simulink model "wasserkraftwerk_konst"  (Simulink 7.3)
settings: Solver=ode23tb  StartTime=0.0  StopTime=1000  MaxStep=0.1  RelTol=1e-4
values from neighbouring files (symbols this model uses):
  A_V0 = 0.518    [Parameter_sim.m]
  A_W = 5^2*pi    (= 78.5398163397)    [Parameter_sim.m]
  c_d = 0.9658    [Parameter_sim.m]
  d_F = 2    [Parameter_sim.m]
  d_T = 3    [Parameter_sim.m]
  d_Turb = 5.35    [Parameter_sim.m]
  g = 9.81    [Parameter_sim.m]
  h_R = 413    [Parameter_sim.m]
  h_W0 = 390    [Parameter_sim.m]
  h_W_IC = 413    [Parameter_sim.m]
  I_IC = 0    [Parameter_sim.m]
  kappa = 8.7*10^3    (= 8700)    [Parameter_sim.m]
  l_F = 741    [Parameter_sim.m]
  L_G = 0.1    [Parameter_sim.m]
  L_net = 0.1    [Parameter_sim.m]
  l_T = 2000    [Parameter_sim.m]
  lambda_F = 0.0153    [Parameter_sim.m]
  lambda_T = 0.0182    [Parameter_sim.m]
  lambda_W = 4.0738    [Parameter_sim.m]
  omega_IC = 0    [Parameter_sim.m]
  p_0 = 0    [Parameter_sim.m]
  R_G = 10    [Parameter_sim.m]
  R_net = 165    [Parameter_sim.m]
  rho = 1000    [Parameter_sim.m]
  sigma_0 = 6.2790e-010    (= 6.279e-10)    [Parameter_sim.m]
  Theta = 5.4997*10^3    (= 5499.7)    [Parameter_sim.m]
  v_F_IC = 0    [Parameter_sim.m]
  V_F_IC = l_F*pi*d_F^2/4    (= 2327.92015631)    [Parameter_sim.m]
  v_T_IC = 0    [Parameter_sim.m]

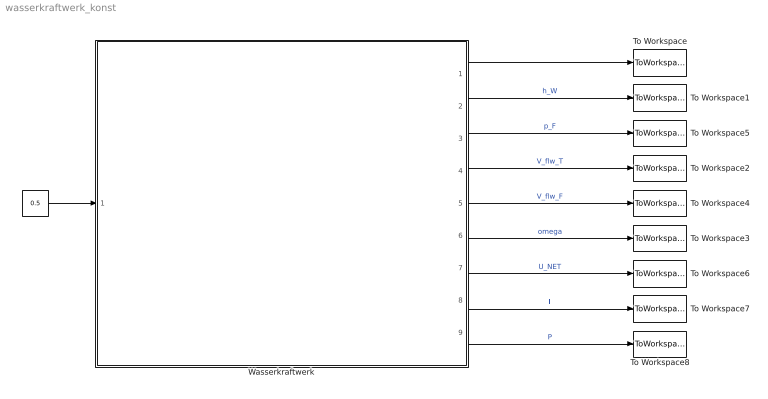
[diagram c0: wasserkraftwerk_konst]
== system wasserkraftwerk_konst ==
  " " : Constant  Value=0.5  OutDataType=sfix(16)  OutScaling=2^0
  To Workspace : ToWorkspace  VariableName=x  SampleTime=-1  SaveFormat=Array
  To Workspace1 : ToWorkspace  VariableName=h_W  SampleTime=-1  SaveFormat=Array
  To Workspace2 : ToWorkspace  VariableName=V_flw_T  SampleTime=-1  SaveFormat=Array
  To Workspace3 : ToWorkspace  VariableName=omega  SampleTime=-1  SaveFormat=Array
  To Workspace4 : ToWorkspace  VariableName=V_flw_F  SampleTime=-1  SaveFormat=Array
  To Workspace5 : ToWorkspace  VariableName=p_F  SampleTime=-1  SaveFormat=Array
  To Workspace6 : ToWorkspace  VariableName=U_NET  SampleTime=-1  SaveFormat=Array
  To Workspace7 : ToWorkspace  VariableName=I  SampleTime=-1  SaveFormat=Array
  To Workspace8 : ToWorkspace  VariableName=P  SampleTime=-1  SaveFormat=Array
  Wasserkraftwerk : Subsystem
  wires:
  " "/1 -> Wasserkraftwerk/1(in)
  Wasserkraftwerk/1(x) -> To Workspace/1
  Wasserkraftwerk/2(h_W) -> To Workspace1/1  "h_W"
  Wasserkraftwerk/3(p_F) -> To Workspace5/1  "p_F"
  Wasserkraftwerk/4(V_flw_T) -> To Workspace2/1  "V_flw_T"
  Wasserkraftwerk/5(V_flw_F) -> To Workspace4/1  "V_flw_F"
  Wasserkraftwerk/6(omega) -> To Workspace3/1  "omega"
  Wasserkraftwerk/7(U_NET) -> To Workspace6/1  "U_NET"
  Wasserkraftwerk/8(I) -> To Workspace7/1  "I"
  Wasserkraftwerk/9(P) -> To Workspace8/1  "P"

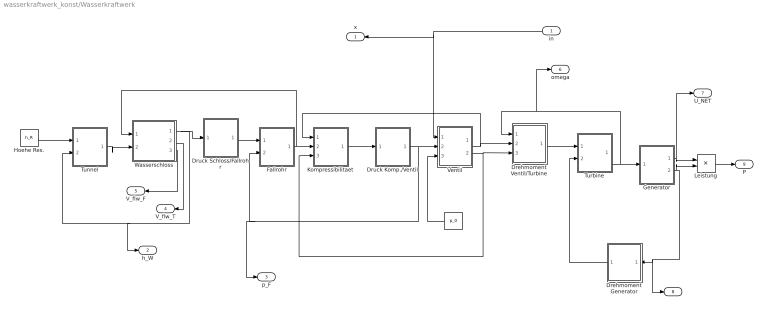
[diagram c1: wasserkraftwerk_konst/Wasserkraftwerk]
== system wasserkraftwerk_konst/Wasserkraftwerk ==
  in : Inport  OutDataType=sfix(16)  OutScaling=2^0
  " " : Constant  Value=p_0  OutDataType=sfix(16)  OutScaling=2^0
  Drehmoment Generator : Subsystem
  Drehmoment Ventil/Turbine : Subsystem
  Druck Komp./Ventil : Subsystem
  Druck Schloss/Fallrohr : Subsystem
  Fallrohr : Subsystem
  Generator : Subsystem
  Hoehe Res. : Constant  Value=h_R  OutDataType=sfix(16)  OutScaling=2^0
  Kompressibilitaet : Subsystem
  Leistung : Product  OutDataType=sfix(16)  OutScaling=2^0
  Tunnel : Subsystem
  Turbine : Subsystem
  Ventil : Subsystem
  Wasserschloss : Subsystem
  x : Outport  OutDataType=sfix(16)  OutScaling=2^0
  h_W : Outport  Port=2  OutDataType=sfix(16)  OutScaling=2^0
  p_F : Outport  Port=3  OutDataType=sfix(16)  OutScaling=2^0
  V_flw_T : Outport  Port=4  OutDataType=sfix(16)  OutScaling=2^0
  V_flw_F : Outport  Port=5  OutDataType=sfix(16)  OutScaling=2^0
  omega : Outport  Port=6  OutDataType=sfix(16)  OutScaling=2^0
  U_NET : Outport  Port=7  OutDataType=sfix(16)  OutScaling=2^0
  I : Outport  Port=8  OutDataType=sfix(16)  OutScaling=2^0
  P : Outport  Port=9  OutDataType=sfix(16)  OutScaling=2^0
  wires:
  Hoehe Res./1 -> Tunnel/1(h_R)
  Tunnel/1(v_T) -> Wasserschloss/2(v_T)
  Wasserschloss/1(h_W) -> Druck Schloss/Fallrohr/1(h_W), Tunnel/2(h_W), h_W/1
  Druck Schloss/Fallrohr/1(p_W) -> Fallrohr/1(p_W)
  Fallrohr/1(v_F) -> Kompressibilitaet/2(v_F), Wasserschloss/1(v_F)
  Kompressibilitaet/1(V) -> Druck Komp./Ventil/1(V)
  Druck Komp./Ventil/1(p_F) -> Ventil/2(p_F), Fallrohr/2(p_F), p_F/1
  Ventil/1(A_V) -> Drehmoment Ventil/Turbine/2(A_V), Kompressibilitaet/1(A_V)
  Drehmoment Ventil/Turbine/1(T_T) -> Turbine/1(T_T)
  Turbine/1(w) -> Generator/1(w), Drehmoment Ventil/Turbine/1(w), omega/1
  Generator/2(I) -> Drehmoment Generator/1(I), I/1, Leistung/2
  Ventil/2(v_V) -> Drehmoment Ventil/Turbine/3(v_V), Kompressibilitaet/3(v_V)
  Generator/1(U_NET) -> U_NET/1, Leistung/1
  Leistung/1 -> P/1
  Wasserschloss/2(V_flw_T) -> V_flw_T/1
  Wasserschloss/3(V_flw_F) -> V_flw_F/1
  " "/1 -> Ventil/3(p_0)
  Drehmoment Generator/1(T_G) -> Turbine/2(T_G)
  in/1 -> Ventil/1(x), x/1

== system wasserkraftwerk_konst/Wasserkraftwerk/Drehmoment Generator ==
  I : Inport  OutDataType=sfix(16)  OutScaling=2^0
  Gain : Gain  Gain=kappa  ParameterDataType=sfix(16)  ParameterScaling=2^0  OutDataType=sfix(16)  OutScaling=2^0
  T_G : Outport  OutDataType=sfix(16)  OutScaling=2^0
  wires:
  I/1 -> Gain/1
  Gain/1 -> T_G/1

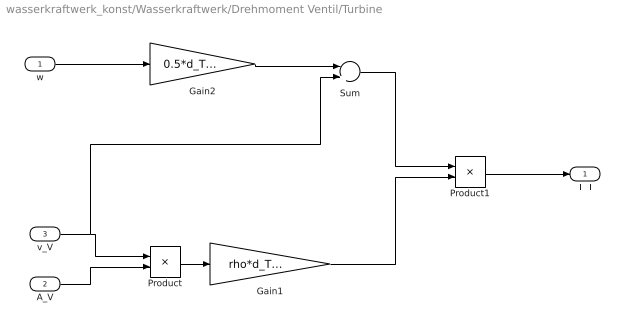
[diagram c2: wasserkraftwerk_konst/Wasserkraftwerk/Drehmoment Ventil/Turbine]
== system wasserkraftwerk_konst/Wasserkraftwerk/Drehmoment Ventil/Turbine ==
  w : Inport  OutDataType=sfix(16)  OutScaling=2^0
  A_V : Inport  Port=2  OutDataType=sfix(16)  OutScaling=2^0
  v_V : Inport  Port=3  OutDataType=sfix(16)  OutScaling=2^0
  Gain1 : Gain  Gain=rho*d_Turb  ParameterDataType=sfix(16)  ParameterScaling=2^0  OutDataType=sfix(16)  OutScaling=2^0
  Gain2 : Gain  Gain=0.5*d_Turb  ParameterDataType=sfix(16)  ParameterScaling=2^0  OutDataType=sfix(16)  OutScaling=2^0
  Product : Product  OutDataType=sfix(16)  OutScaling=2^0
  Product1 : Product  OutDataType=sfix(16)  OutScaling=2^0
  Sum : Sum  Inputs=-+  OutDataType=sfix(16)  OutScaling=2^0
  T_T : Outport  OutDataType=sfix(16)  OutScaling=2^0
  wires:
  Product/1 -> Gain1/1
  w/1 -> Gain2/1
  Gain2/1 -> Sum/1
  v_V/1 -> Product/1, Sum/2
  A_V/1 -> Product/2
  Sum/1 -> Product1/1
  Gain1/1 -> Product1/2
  Product1/1 -> T_T/1

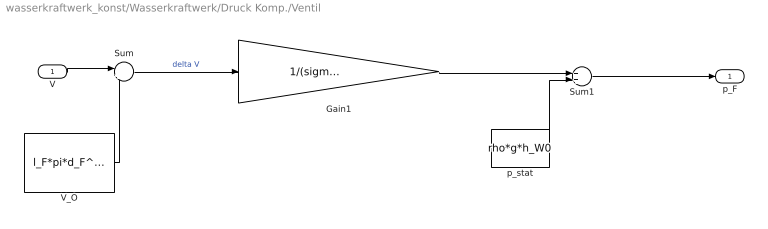
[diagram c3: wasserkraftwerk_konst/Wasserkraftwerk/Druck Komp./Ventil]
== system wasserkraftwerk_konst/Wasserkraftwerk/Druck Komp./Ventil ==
  V : Inport  OutDataType=sfix(16)  OutScaling=2^0
  Gain1 : Gain  Gain=1/(sigma_0 * l_F*pi*d_F^2/4)  ParameterDataType=sfix(16)  ParameterScaling=2^0  OutDataType=sfix(16)  OutScaling=2^0
  Sum : Sum  Inputs=|+-  OutDataType=sfix(16)  OutScaling=2^0
  Sum1 : Sum  OutDataType=sfix(16)  OutScaling=2^0
  V_O : Constant  Value=l_F*pi*d_F^2/4  OutDataType=sfix(16)  OutScaling=2^0
  p_stat : Constant  Value=rho*g*h_W0  OutDataType=sfix(16)  OutScaling=2^0
  p_F : Outport  OutDataType=sfix(16)  OutScaling=2^0
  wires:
  V/1 -> Sum/1
  V_O/1 -> Sum/2
  Sum1/1 -> p_F/1
  p_stat/1 -> Sum1/2
  Sum/1 -> Gain1/1  "delta V"
  Gain1/1 -> Sum1/1

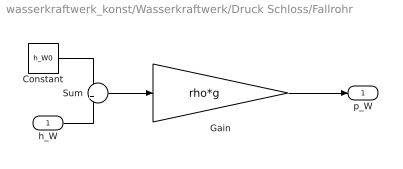
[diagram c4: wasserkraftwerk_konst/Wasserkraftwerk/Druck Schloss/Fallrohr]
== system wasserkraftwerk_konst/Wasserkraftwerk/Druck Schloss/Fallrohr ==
  h_W : Inport  OutDataType=sfix(16)  OutScaling=2^0
  Constant : Constant  Value=h_W0  OutDataType=sfix(16)  OutScaling=2^0
  Gain : Gain  Gain=rho*g  ParameterDataType=sfix(16)  ParameterScaling=2^0  OutDataType=sfix(16)  OutScaling=2^0
  Sum : Sum  Inputs=-+  OutDataType=sfix(16)  OutScaling=2^0
  p_W : Outport  OutDataType=sfix(16)  OutScaling=2^0
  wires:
  Gain/1 -> p_W/1
  Constant/1 -> Sum/1
  h_W/1 -> Sum/2
  Sum/1 -> Gain/1

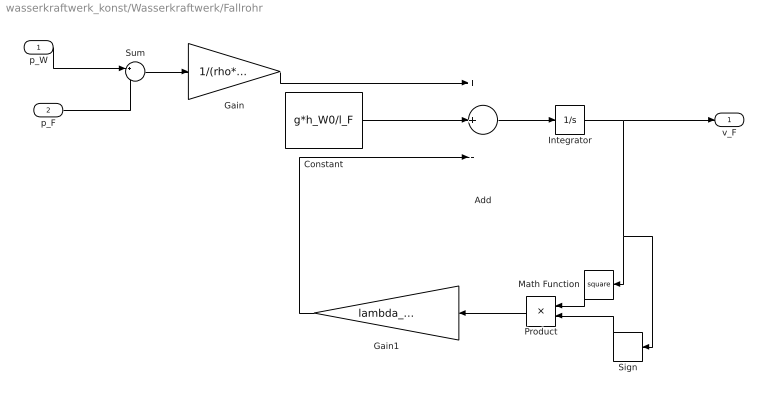
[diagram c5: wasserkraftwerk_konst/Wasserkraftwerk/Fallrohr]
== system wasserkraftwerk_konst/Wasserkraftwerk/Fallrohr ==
  p_W : Inport  OutDataType=sfix(16)  OutScaling=2^0
  p_F : Inport  Port=2  OutDataType=sfix(16)  OutScaling=2^0
  Add : Sum  Inputs=++-  OutDataType=sfix(16)  OutScaling=2^-10
  Constant : Constant  Value=g*h_W0/l_F  OutDataType=sfix(16)  OutScaling=2^0
  Gain : Gain  Gain=1/(rho*l_F)  ParameterDataType=sfix(16)  ParameterScaling=2^0  OutDataType=sfix(16)  OutScaling=2^0
  Gain1 : Gain  Gain=lambda_F/(2*d_F)  ParameterDataType=sfix(16)  ParameterScaling=2^0  OutDataType=sfix(16)  OutScaling=2^0
  Integrator : Integrator  InitialCondition=v_F_IC
  Math Function : Math  Operator=square  OutDataType=sfix(16)  OutScaling=2^0
  Product : Product  OutDataType=sfix(16)  OutScaling=2^0
  Sign : Signum
  Sum : Sum  Inputs=+-  OutDataType=sfix(16)  OutScaling=2^0
  v_F : Outport  OutDataType=sfix(16)  OutScaling=2^0
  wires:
  Product/1 -> Gain1/1
  Sign/1 -> Product/2
  p_W/1 -> Sum/1
  p_F/1 -> Sum/2
  Sum/1 -> Gain/1
  Gain/1 -> Add/1
  Gain1/1 -> Add/3
  Add/1 -> Integrator/1
  Integrator/1 -> v_F/1, Math Function/1, Sign/1
  Math Function/1 -> Product/1
  Constant/1 -> Add/2

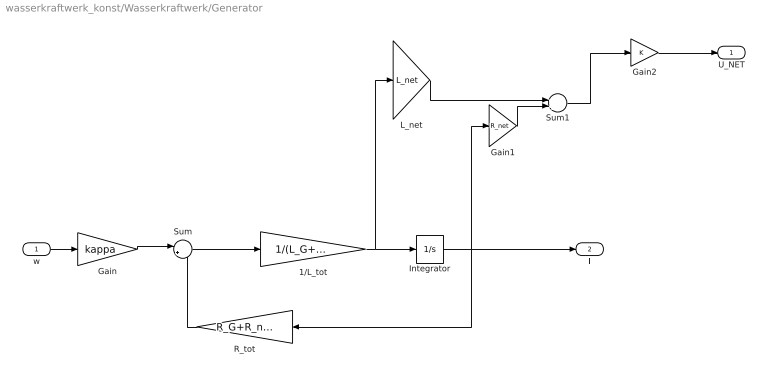
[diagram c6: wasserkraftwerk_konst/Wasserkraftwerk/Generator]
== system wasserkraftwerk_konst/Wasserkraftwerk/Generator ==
  w : Inport  OutDataType=sfix(16)  OutScaling=2^0
  1/L_tot : Gain  Gain=1/(L_G+L_net)  ParameterDataType=sfix(16)  ParameterScaling=2^0  OutDataType=sfix(16)  OutScaling=2^0
  Gain : Gain  Gain=kappa  ParameterDataType=sfix(16)  ParameterScaling=2^0  OutDataType=sfix(16)  OutScaling=2^0
  Gain1 : Gain  Gain=R_net  ParameterDataType=sfix(16)  ParameterScaling=2^0  OutDataType=sfix(16)  OutScaling=2^0
  Gain2 : Gain  ParameterDataType=sfix(16)  ParameterScaling=2^0  OutDataType=sfix(16)  OutScaling=2^0
  Integrator : Integrator  InitialCondition=I_IC
  L_net : Gain  Gain=L_net  ParameterDataType=sfix(16)  ParameterScaling=2^0  OutDataType=sfix(16)  OutScaling=2^0
  R_tot : Gain  Gain=R_G+R_net  ParameterDataType=sfix(16)  ParameterScaling=2^0  OutDataType=sfix(16)  OutScaling=2^0
  Sum : Sum  Inputs=|+-  OutDataType=sfix(16)  OutScaling=2^0
  Sum1 : Sum  OutDataType=sfix(16)  OutScaling=2^0
  U_NET : Outport  OutDataType=sfix(16)  OutScaling=2^0
  I : Outport  Port=2  OutDataType=sfix(16)  OutScaling=2^0
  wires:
  Integrator/1 -> I/1, R_tot/1, Gain1/1
  w/1 -> Gain/1
  Gain/1 -> Sum/1
  Sum/1 -> 1/L_tot/1
  1/L_tot/1 -> Integrator/1, L_net/1
  Gain2/1 -> U_NET/1
  Gain1/1 -> Sum1/2
  R_tot/1 -> Sum/2
  Sum1/1 -> Gain2/1
  L_net/1 -> Sum1/1

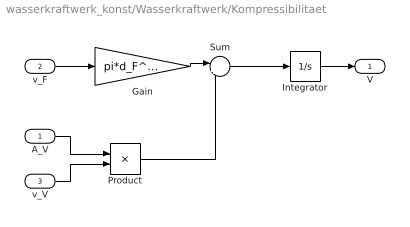
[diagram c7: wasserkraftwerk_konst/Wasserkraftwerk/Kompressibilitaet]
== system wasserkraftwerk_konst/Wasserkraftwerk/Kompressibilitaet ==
  A_V : Inport  OutDataType=sfix(16)  OutScaling=2^0
  v_F : Inport  Port=2  OutDataType=sfix(16)  OutScaling=2^0
  v_V : Inport  Port=3  OutDataType=sfix(16)  OutScaling=2^0
  Gain : Gain  Gain=pi*d_F^2/4  ParameterDataType=sfix(16)  ParameterScaling=2^0  OutDataType=sfix(16)  OutScaling=2^0
  Integrator : Integrator  InitialCondition=V_F_IC
  Product : Product  OutDataType=sfix(16)  OutScaling=2^0
  Sum : Sum  Inputs=|+-  OutDataType=sfix(16)  OutScaling=2^0
  V : Outport  OutDataType=sfix(16)  OutScaling=2^0
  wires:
  v_F/1 -> Gain/1
  Gain/1 -> Sum/1
  A_V/1 -> Product/1
  v_V/1 -> Product/2
  Product/1 -> Sum/2
  Sum/1 -> Integrator/1
  Integrator/1 -> V/1

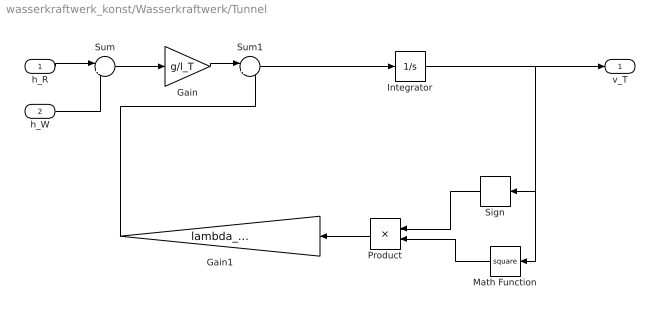
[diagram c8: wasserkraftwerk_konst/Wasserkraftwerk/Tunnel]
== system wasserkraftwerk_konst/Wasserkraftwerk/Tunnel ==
  h_R : Inport  OutDataType=sfix(16)  OutScaling=2^0
  h_W : Inport  Port=2  OutDataType=sfix(16)  OutScaling=2^0
  Gain : Gain  Gain=g/l_T  ParameterDataType=sfix(16)  ParameterScaling=2^0  OutDataType=sfix(16)  OutScaling=2^0
  Gain1 : Gain  Gain=lambda_T/(2*d_T)  ParameterDataType=sfix(16)  ParameterScaling=2^0  OutDataType=sfix(16)  OutScaling=2^0
  Integrator : Integrator  InitialCondition=v_T_IC
  Math Function : Math  Operator=square  OutDataType=sfix(16)  OutScaling=2^0
  Product : Product  OutDataType=sfix(16)  OutScaling=2^0
  Sign : Signum
  Sum : Sum  Inputs=|+-  OutDataType=sfix(16)  OutScaling=2^0
  Sum1 : Sum  Inputs=|+-  OutDataType=sfix(16)  OutScaling=2^0
  v_T : Outport  OutDataType=sfix(16)  OutScaling=2^0
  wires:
  h_R/1 -> Sum/1
  h_W/1 -> Sum/2
  Sum/1 -> Gain/1
  Gain/1 -> Sum1/1
  Sum1/1 -> Integrator/1
  Integrator/1 -> v_T/1, Sign/1, Math Function/1
  Product/1 -> Gain1/1
  Sign/1 -> Product/1
  Math Function/1 -> Product/2
  Gain1/1 -> Sum1/2

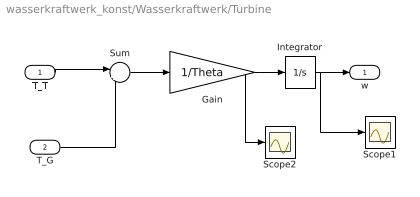
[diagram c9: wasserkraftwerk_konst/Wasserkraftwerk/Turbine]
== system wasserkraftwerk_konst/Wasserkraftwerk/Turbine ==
  T_T : Inport  OutDataType=sfix(16)  OutScaling=2^0
  T_G : Inport  Port=2  OutDataType=sfix(16)  OutScaling=2^0
  Gain : Gain  Gain=1/Theta  ParameterDataType=sfix(16)  ParameterScaling=2^0  OutDataType=sfix(16)  OutScaling=2^0
  Integrator : Integrator  InitialCondition=omega_IC
  Scope1 : Scope
  Scope2 : Scope
  Sum : Sum  Inputs=|+-  OutDataType=sfix(16)  OutScaling=2^0
  w : Outport  OutDataType=sfix(16)  OutScaling=2^0
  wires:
  T_T/1 -> Sum/1
  T_G/1 -> Sum/2
  Sum/1 -> Gain/1
  Gain/1 -> Integrator/1, Scope2/1
  Integrator/1 -> w/1, Scope1/1

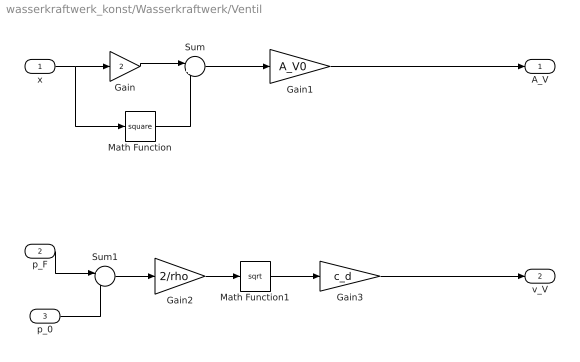
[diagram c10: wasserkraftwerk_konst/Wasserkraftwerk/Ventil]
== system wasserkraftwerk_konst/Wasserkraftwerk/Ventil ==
  x : Inport  OutDataType=sfix(16)  OutScaling=2^0
  p_F : Inport  Port=2  OutDataType=sfix(16)  OutScaling=2^0
  p_0 : Inport  Port=3  OutDataType=sfix(16)  OutScaling=2^0
  Gain : Gain  Gain=2  ParameterDataType=sfix(16)  ParameterScaling=2^0  OutDataType=sfix(16)  OutScaling=2^0
  Gain1 : Gain  Gain=A_V0  ParameterDataType=sfix(16)  ParameterScaling=2^0  OutDataType=sfix(16)  OutScaling=2^0
  Gain2 : Gain  Gain=2/rho  ParameterDataType=sfix(16)  ParameterScaling=2^0  OutDataType=sfix(16)  OutScaling=2^0
  Gain3 : Gain  Gain=c_d  ParameterDataType=sfix(16)  ParameterScaling=2^0  OutDataType=sfix(16)  OutScaling=2^0
  Math Function : Math  Operator=square  OutDataType=sfix(16)  OutScaling=2^0
  Math Function1 : Math  Operator=sqrt  OutDataType=sfix(16)  OutScaling=2^0
  Sum : Sum  Inputs=|+-  OutDataType=sfix(16)  OutScaling=2^0
  Sum1 : Sum  Inputs=+-  OutDataType=sfix(16)  OutScaling=2^0
  A_V : Outport  OutDataType=sfix(16)  OutScaling=2^0
  v_V : Outport  Port=2  OutDataType=sfix(16)  OutScaling=2^0
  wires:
  x/1 -> Gain/1, Math Function/1
  Gain/1 -> Sum/1
  Math Function/1 -> Sum/2
  Sum/1 -> Gain1/1
  Gain1/1 -> A_V/1
  p_F/1 -> Sum1/1
  p_0/1 -> Sum1/2
  Sum1/1 -> Gain2/1
  Gain2/1 -> Math Function1/1
  Math Function1/1 -> Gain3/1
  Gain3/1 -> v_V/1

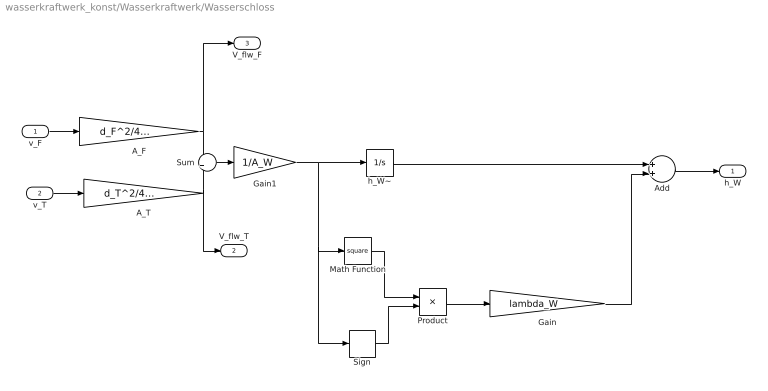
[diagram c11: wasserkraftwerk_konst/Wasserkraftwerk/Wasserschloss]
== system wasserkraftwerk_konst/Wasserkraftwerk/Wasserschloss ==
  v_F : Inport  OutDataType=sfix(16)  OutScaling=2^0
  v_T : Inport  Port=2  OutDataType=sfix(16)  OutScaling=2^0
  A_F : Gain  Gain=d_F^2/4*pi  ParameterDataType=sfix(16)  ParameterScaling=2^0  OutDataType=sfix(16)  OutScaling=2^0
  A_T : Gain  Gain=d_T^2/4*pi  ParameterDataType=sfix(16)  ParameterScaling=2^0  OutDataType=sfix(16)  OutScaling=2^0
  Add : Sum  OutDataType=sfix(16)  OutScaling=2^-10
  Gain : Gain  Gain=lambda_W  ParameterDataType=sfix(16)  ParameterScaling=2^0  OutDataType=sfix(16)  OutScaling=2^0
  Gain1 : Gain  Gain=1/A_W  ParameterDataType=sfix(16)  ParameterScaling=2^0  OutDataType=sfix(16)  OutScaling=2^0
  Math Function : Math  Operator=square  OutDataType=sfix(16)  OutScaling=2^0
  Product : Product  OutDataType=sfix(16)  OutScaling=2^0
  Sign : Signum
  Sum : Sum  Inputs=-+  OutDataType=sfix(16)  OutScaling=2^0
  h_W~ : Integrator  InitialCondition=h_W_IC
  h_W : Outport  OutDataType=sfix(16)  OutScaling=2^0
  V_flw_T : Outport  Port=2  OutDataType=sfix(16)  OutScaling=2^0
  V_flw_F : Outport  Port=3  OutDataType=sfix(16)  OutScaling=2^0
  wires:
  Product/1 -> Gain/1
  v_T/1 -> A_T/1
  v_F/1 -> A_F/1
  A_F/1 -> Sum/1, V_flw_F/1
  A_T/1 -> Sum/2, V_flw_T/1
  Sum/1 -> Gain1/1
  Gain1/1 -> h_W~/1, Math Function/1, Sign/1
  Math Function/1 -> Product/1
  Sign/1 -> Product/2
  h_W~/1 -> Add/1
  Add/1 -> h_W/1
  Gain/1 -> Add/2
